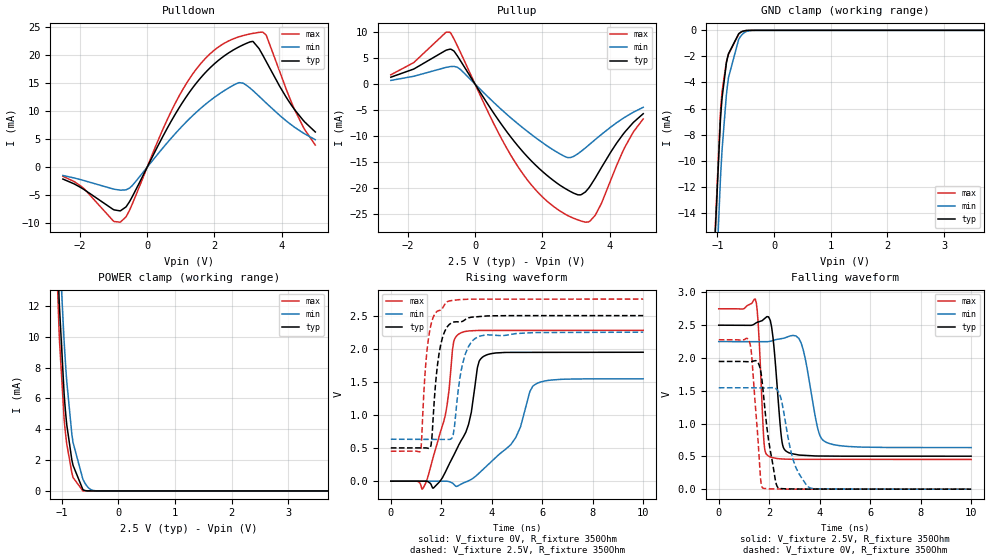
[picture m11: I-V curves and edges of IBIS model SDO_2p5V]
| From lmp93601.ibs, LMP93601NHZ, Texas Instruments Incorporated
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|   Model SDO_2p5V
[Model]   SDO_2p5V
Model_type   3-state
Polarity   Non-Inverting
Vmeas = 1.25
Vref = 2.5
Cref = 15pF
Rref = 350
|   typ   min   max
|   (nom PVT)   (fast PVT)   (slow PVT)
C_comp   0.1400p   0.1309p   0.1458p
|C_comp (ON state)   0.1476p   0.1455p   0.1492p
|C_comp (OFF state)   0.1400p   0.1309p   0.1458p
[Voltage Range]   2.5   2.25   2.75
[Temperature Range]   27   125   -25
[Pullup Reference]   2.5   2.25   2.75
[Pulldown Reference]   0   0   0
[Power Clamp Reference]   2.5   2.25   2.75
[GND Clamp Reference]   0   0   0
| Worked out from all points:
|   slope of the pulldown table from 0 to 0.375 V, typ, clamps not added: 84.4 ohm
|   slope of the pullup table from 0 to 0.375 V, typ, clamps not added: 98.3 ohm
|   GND clamp passes 1 mA (typ) near -0.71 V on its own axis
|   POWER clamp passes 1 mA (typ) near -0.73 V on its own axis
|   falling waveform, V_fixture 2.5V, R_fixture 350Ohm: 20-80 % time 249ps typ, 445ps min, 165ps max; typ from 2.5 V to 0.502 V
|   rising waveform, V_fixture 0V, R_fixture 350Ohm: 20-80 % time 885ps typ, 1.41ns min, 659ps max; typ from 0 V to 1.95 V
|   rising waveform, V_fixture 2.5V, R_fixture 350Ohm: 20-80 % time 334ps typ, 402ps min, 297ps max; typ from 0.502 V to 2.5 V
|   falling waveform, V_fixture 0V, R_fixture 350Ohm: 20-80 % time 395ps typ, 537ps min, 258ps max; typ from 1.95 V to 0 V
[Pulldown]
|   Voltage   I(typ)   I(min)   I(max)
-2.5V     -2.092mA   -1.454mA   -1.603mA
-790mV    -7.737mA   -4.077mA   -9.736mA
-520mV    -6.101mA   -3.696mA   -7.633mA
740mV     8.473mA    5.35mA     10.27mA
1.407V    14.58mA    9.509mA    17.06mA
2V        18.44mA    12.46mA    20.88mA
2.72V     21.42mA    15.05mA    23.22mA
3.125V    22.41mA    13.75mA    23.82mA
3.328V    21.08mA    12.63mA    24.03mA
3.545V    18.73mA    11.38mA    23.38mA
4.378V    10.27mA    7.132mA    10.29mA
4.992V    6.287mA    4.91mA     3.957mA
[GND Clamp]
|   Voltage   I(typ)   I(min)   I(max)
-2.5V     -338mA     -305.4mA   -363.8mA
-1.038V   -15.45mA   -20.64mA   -15.05mA
-947.5mV  -6.899mA   -11.43mA   -6.287mA
-940mV    -6.416mA   -10.81mA   -5.831mA
-917.5mV  -5.153mA   -9.12mA    -4.673mA
-842.5mV  -2.523mA   -4.971mA   -2.434mA
-805mV    -1.795mA   -3.622mA   -1.836mA
-625mV    -267uA     -693.8uA   -290uA
-565mV    -94.34uA   -328.7uA   -89.26uA
-475mV    -11.95uA   -68.91uA   -8.046uA
-310mV    -98.22nA   -1.584uA   -24.86nA
4.992V    0A         0A         0A
[Pullup]
|   Voltage   I(typ)   I(min)   I(max)
-2.5V     1.318mA    699.7uA    1.775mA
-1.817V   2.887mA    1.499mA    4.133mA
-745mV    6.696mA    3.341mA    9.933mA
-437.5mV  4.53mA     2.825mA    6.14mA
635mV     -6.345mA   -4.001mA   -8.612mA
1.423V    -13.01mA   -8.408mA   -17.25mA
2V        -16.77mA   -11.24mA   -21.65mA
2.735V    -20.27mA   -14.08mA   -25.18mA
3.275V    -20.71mA   -12.26mA   -26.51mA
3.575V    -17.97mA   -10.62mA   -25.1mA
4.445V    -9.228mA   -6.374mA   -12.14mA
4.992V    -5.69mA    -4.462mA   -6.687mA
[POWER Clamp]
|   Voltage   I(typ)   I(min)   I(max)
-2.5V     222.8mA    201.7mA    237mA
-1.135V   21.68mA    24.75mA    19.94mA
-1.045V   12.55mA    16.34mA    10.38mA
-1.038V   11.9mA     15.71mA    9.742mA
-955mV    6.271mA    9.661mA    4.639mA
-910mV    4.315mA    7.137mA    3.068mA
-820mV    2.025mA    3.706mA    1.192mA
-797.5mV  1.655mA    3.131mA    866.1uA
-625mV    92.08uA    761uA      6.15uA
-512.5mV  2.045uA    160.4uA    151.8nA
-370mV    9.915nA    4.839uA    0A
4.992V    0A         0A         0A
[Ramp]
R_load = 350
|   typ   min   max
dV/dt_r   1.16817/8.84912e-10   0.927462/1.40501e-09   1.36656/6.58758e-10
dV/dt_f   1.1985/2.49001e-10   0.969808/4.44514e-10   1.37829/1.64729e-10
[Falling Waveform]
V_fixture = 2.5V
V_fixture_min = 2.25V
V_fixture_max = 2.75V
R_fixture = 350Ohm
C_fixture = 0F
|   Time   V(typ)   V(min)   V(max)
0s        2.5V       2.25V      2.75V
1.45ns    2.527V     2.249V     2.898V
1.797ns   2.594V     2.248V     696.3mV
1.96ns    2.628V     2.249V     507.1mV
2.146ns   2.326V     2.266V     480.1mV
2.482ns   794.3mV    2.295V     461.5mV
2.7ns     570.9mV    2.318V     457.6mV
3.264ns   518.4mV    2.23V      454.9mV
4.186ns   504.9mV    730.4mV    454.6mV
10ns      502.5mV    633.7mV    452.9mV
[Rising Waveform]
V_fixture = 0V
V_fixture_min = 0V
V_fixture_max = 0V
R_fixture = 350Ohm
C_fixture = 0F
|   Time   V(typ)   V(min)   V(max)
0s        3.619nV    11.93nV    5.073nV
1.37ns    494.6uV    15.74uV    -39.31mV
2.155ns   132.9mV    24.76uV    989.5mV
2.492ns   391mV      -45.17mV   2.108V
2.689ns   544.4mV    -64.11mV   2.221V
3.083ns   861.1mV    6.457mV    2.269V
3.696ns   1.889V     193mV      2.276V
4.953ns   1.945V     659.9mV    2.277V
5.716ns   1.945V     1.46V      2.277V
10ns      1.947V     1.546V     2.278V
[Rising Waveform]
V_fixture = 2.5V
V_fixture_min = 2.25V
V_fixture_max = 2.75V
R_fixture = 350Ohm
C_fixture = 0F
|   Time   V(typ)   V(min)   V(max)
0s        502.5mV    633.7mV    452.9mV
1.18ns    502.8mV    631.8mV    459.5mV
1.37ns    502.8mV    631.5mV    1.697V
1.562ns   507.7mV    631.2mV    2.313V
1.908ns   1.92V      630.7mV    2.576V
2.226ns   2.324V     630.2mV    2.708V
2.472ns   2.401V     700.2mV    2.73V
2.95ns    2.44V      1.919V     2.746V
3.461ns   2.484V     2.181V     2.748V
10ns      2.5V       2.25V      2.75V
[Falling Waveform]
|Gnd
V_fixture = 0V
V_fixture_min = 0V
V_fixture_max = 0V
R_fixture = 350Ohm
C_fixture = 0F
|   Time   V(typ)   V(min)   V(max)
0s        1.947V     1.546V     2.278V
1.237ns   1.943V     1.546V     2.218V
1.594ns   1.899V     1.544V     529.4mV
1.664ns   1.799V     1.544V     139.5mV
1.749ns   1.533V     1.543V     15.91mV
1.976ns   742mV      1.545V     5.675mV
2.37ns    17.71mV    1.481V     2.455mV
2.95ns    3.267mV    444.6mV    688.4uV
3.575ns   1.164mV    28.83mV    627.4uV
10ns      69.27nV    817nV      497.6nV
